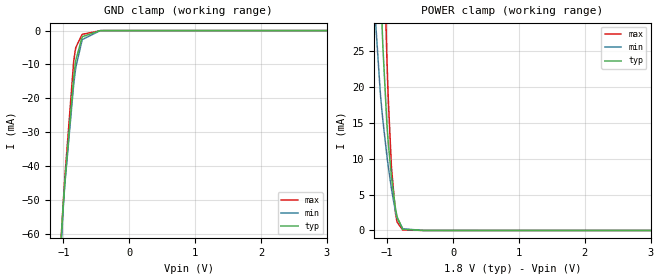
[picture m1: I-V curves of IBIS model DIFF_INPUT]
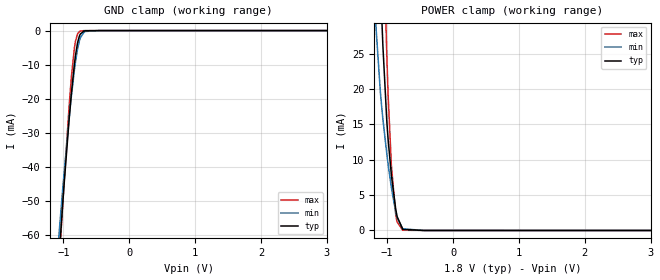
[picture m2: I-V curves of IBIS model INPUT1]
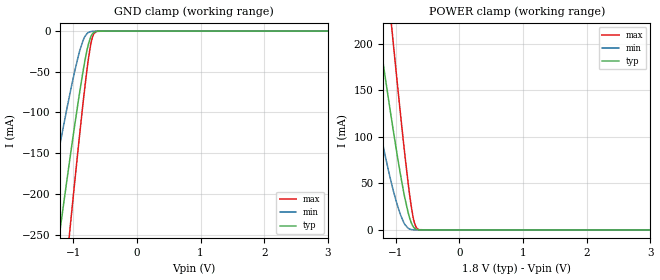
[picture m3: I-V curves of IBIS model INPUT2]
|Texas Instruments Incorporated
|FPD-Link III 4.16 Gbps Serializer w/CSI-2 interface for 2.3MP/60fps cameras
|Marketing part#   Digital Voltage Range   Package-type   #pins
|DS90UB953A-Q1   1.71V to 1.89V   QFN   32
[IBIS Ver]   4.1
[File name]   ds90ub953a-q1.ibs
[File Rev]   1.0
[Date]   03/19/19
[Source]
| Texas Instruments Incorporated.
| Analog-eLab Design Center, HPA
| 12500 TI Blvd
| Dallas, TX -75243
[Notes]   Revision History:
| Rev 1.0: 03/19/19
| - Initial version of the model
| - Model generated from simulations in SPECTRE
| - Model matched to SPICE simulation
| - C_comp although listed in numerical order of value are
|   obtained from varying PVT conditions. For PVT conditions for
|   each specific value refer the buffer description under
|   respective [Model]. IBIS model user is responsible for using
|   appropriate C_comp to simulate for Signal Integrity.
|* EXCEPTION:*
|*  Differential output pins (DIFF_OUT) can operate with bit rate of 4.16Gbps (or 2.08GHz frequency).
|   However, due to IV-VT mismatches >2.2% in SIMDE for higher frequencies,
|   DIFF_OUT IBIS model is generated at frequency of 250MHz or 500Mbps bit rate.
|*  For DIFF_OUT, VT curves were exacted with delay adjustment so that all three corner's
|   rising and falling edges will align around the same time.
|   Also, initial flat response of 170ps has been removed in VT curves (both rising and falling).
|*  INPUT3 IBIS model corresponds to TDI, TCK, TMS pins which are present in design,
|   but not mentioned in the data-sheet.
|*  TDO pin's (present in schematic design) buffer is similar to that of GPIO's.
|   So, for TDO, GPIO model can be used.
[Disclaimer]
| This model is designed as an aid for customers of Texas Instruments.
| TI and its licensors and suppliers make no warranties, either expressed
| or implied, with respect to this  model, including the warranties of
| merchantability or fitness for a particular purpose. The model is
| provided solely on an "as is" basis. The entire risk as to its quality
| and performance is with the customer.
[Copyright]
(C) Copyright 2019 Texas Instruments Incorporated.All rights reserved.
|   DS90UB953A-Q1
[Component]   DS90UB953A-Q1
[Manufacturer]   TI
[Package]   |QFN (32)
|   typ   min   max
R_pkg   0.067   0.027   0.083
L_pkg   0.937nH   0.593nH   1.143nH
C_pkg   0.144pF   0.126pF   0.200pF
[Pin]  signal_name   model_name   R_pin   L_pin   C_pin
1   CSI_D1P   DIFF_INPUT   NA   NA   NA
2   CSI_D1N   DIFF_INPUT   NA   NA   NA
3   CSI_D0P   DIFF_INPUT   NA   NA   NA
4   CSI_D0N   DIFF_INPUT   NA   NA   NA
5   CSI_CLKP   DIFF_INPUT   NA   NA   NA
6   CSI_CLKN   DIFF_INPUT   NA   NA   NA
7   RES0   nc   NA   NA   NA
8   PDB   INPUT1   NA   NA   NA
9   LPF1   nc   NA   NA   NA
10   VDDPLL_CAP   power   NA   NA   NA
11   VDDPLL   power   NA   NA   NA
12   LPF2   nc   NA   NA   NA
13   DOUTN   DIFF_OUT   NA   NA   NA
14   DOUTP   DIFF_OUT   NA   NA   NA
15   VDDRV_CAP   power   NA   NA   NA
16   VDDRV   power   NA   NA   NA
17   GPIO_0   GPIO   NA   NA   NA
18   GPIO_1   GPIO   NA   NA   NA
19   CLK_OUT/IDx   GPIO   NA   NA   NA
20   CLKIN   GPIO   NA   NA   NA
21   MODE   INPUT2   NA   NA   NA
22   RES1   nc   NA   NA   NA
23   I2C_SDA   IO_OPEN_DRAIN   NA   NA   NA
24   I2C_SCL   IO_OPEN_DRAIN   NA   NA   NA
25   VDDD   power   NA   NA   NA
26   VDD_CAP   power   NA   NA   NA
27   GPIO_2   GPIO   NA   NA   NA
28   GPIO_3   GPIO   NA   NA   NA
29   CSI_D3P   DIFF_INPUT   NA   NA   NA
30   CSI_D3N   DIFF_INPUT   NA   NA   NA
31   CSI_D2P   DIFF_INPUT   NA   NA   NA
32   CSI_D2N   DIFF_INPUT   NA   NA   NA
| Models and submodels in the file (7): DIFF_INPUT (Input), INPUT1 (Input), INPUT2 (Input), INPUT3 (Input), GPIO (I/O), IO_OPEN_DRAIN (I/O_open_drain), DIFF_OUT (Output)
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|   DIFF_INPUT Model
[Model]   DIFF_INPUT
Model_type   Input
Vinl = 0.63
Vinh = 1.17
|   typ   min   max
C_comp   0.643pF   0.2943pF   1.006pF
| Where Nom  PVT is Nominal Process, 1.8V, 27C
|   Fast PVT is Strong Process,  1.89V, -40C
|   Slow PVT is Weak Process,   1.71V, 105C
[Model spec]
|subparameter
Vinl   0.63   0.5985   0.6615
Vinh   1.17   1.1115   1.2285
[Voltage Range]   1.8   1.71   1.89
|Junction Temperature
[Temperature Range]   27   105   -40
[Power Clamp Reference]   1.8   1.71   1.89
[GND Clamp Reference]   0   0   0
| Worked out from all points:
|   POWER clamp passes 1 mA (typ) near -0.81 V on its own axis
[GND Clamp]
|   Voltage   I(typ)   I(min)   I(max)
-1.8V     -624.4mA   -649mA     -608.7mA
-1.098V   -81.74mA   -87.49mA   -82.03mA
-1.006V   -52.48mA   -53.16mA   -51.77mA
-979.2mV  -44.98mA   -45.4mA    -43.38mA
-844.2mV  -13.86mA   -15.81mA   -9.084mA
-822.6mV  -10.25mA   -12.35mA   -6.067mA
-811.8mV  -8.685mA   -10.79mA   -4.955mA
-714.6mV  -1.816mA   -2.648mA   -1.108mA
-444.6mV  -17.03uA   -18.94uA   -49.75uA
3.6V      0A         0A         0A
[POWER Clamp]
|   Voltage   I(typ)   I(min)   I(max)
-1.8V     331.9mA    249.9mA    400.2mA
-1.179V   59.49mA    29.36mA    93.17mA
-1.103V   35.12mA    19.01mA    60.1mA
-1.076V   28.11mA    16.31mA    49.14mA
-1.066V   25.62mA    15.32mA    44.93mA
-1.006V   15.06mA    10.52mA    24.47mA
-984.6mV  12.32mA    8.971mA    18.54mA
-936mV    7.498mA    5.817mA    8.867mA
-876.6mV  3.248mA    2.737mA    2.61mA
-849.6mV  1.896mA    1.725mA    1.174mA
-763.2mV  150.9uA    233uA      49.83uA
3.6V      0A         0A         0A
|   INPUT1 Model
[Model]   INPUT1
Model_type   Input
Vinl = 0.63
Vinh = 1.17
|   typ   min   max
C_comp   1.419pF   1.393pF   1.424pF
| Where Nom  PVT is Nominal Process, 1.8V, 27C
|   Fast PVT is Strong Process,  1.89V, -40C
|   Slow PVT is Weak Process,   1.71V, 105C
[Model spec]
|subparameter
Vinl   0.63   0.5985   0.6615
Vinh   1.17   1.1115   1.2285
[Voltage Range]   1.8   1.71   1.89
|Junction Temperature
[Temperature Range]   27   105   -40
[Power Clamp Reference]   1.8   1.71   1.89
[GND Clamp Reference]   0   0   0
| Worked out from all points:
|   GND clamp passes 1 mA (typ) near -0.74 V on its own axis
|   POWER clamp passes 1 mA (typ) near -0.80 V on its own axis
[GND Clamp]
|   Voltage   I(typ)   I(min)   I(max)
-1.8V     -298mA     -267.8mA   -325mA
-1.06V    -64.74mA   -58.15mA   -66.91mA
-1.012V   -51.07mA   -46.73mA   -51.25mA
-914.4mV  -26.27mA   -25.96mA   -22.47mA
-876.6mV  -17.95mA   -18.79mA   -13.12mA
-833.4mV  -9.837mA   -11.56mA   -5.07mA
-817.2mV  -7.329mA   -9.21mA    -3.105mA
-784.8mV  -3.504mA   -5.314mA   -940.8uA
-752.4mV  -1.371mA   -2.661mA   -231.5uA
-666mV    -62.37uA   -251.7uA   -4.974uA
-444.6mV  -453.1nA   -613.8nA   -563.7nA
3.6V      0A         0A         0A
[POWER Clamp]
|   Voltage   I(typ)   I(min)   I(max)
-1.8V     333.1mA    250.9mA    401.5mA
-1.179V   60.1mA     29.95mA    93.71mA
-1.103V   35.67mA    19.51mA    60.56mA
-1.076V   28.64mA    16.77mA    49.57mA
-1.066V   26.14mA    15.76mA    45.35mA
-1.006V   15.49mA    10.85mA    24.82mA
-984.6mV  12.71mA    9.259mA    18.86mA
-936mV    7.769mA    6.018mA    9.098mA
-871.2mV  3.069mA    2.609mA    2.33mA
-849.6mV  1.979mA    1.793mA    1.201mA
-763.2mV  150uA      234.3uA    33.25uA
3.6V      0A         0A         0A
|   INPUT2 Model
[Model]   INPUT2
Model_type   Input
Vinl = 0.63
Vinh = 1.17
|   typ   min   max
C_comp   0.6431pF   0.2942pF   1.006pF
| Where Nom  PVT is Nominal Process, 1.8V, 27C
|   Fast PVT is Strong Process,  1.89V, -40C
|   Slow PVT is Weak Process,   1.71V, 105C
[Model spec]
|subparameter
Vinl   0.63   0.5985   0.6615
Vinh   1.17   1.1115   1.2285
[Voltage Range]   1.8   1.71   1.89
|Junction Temperature
[Temperature Range]   27   105   -40
[Power Clamp Reference]   1.8   1.71   1.89
[GND Clamp Reference]   0   0   0
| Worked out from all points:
|   GND clamp passes 1 mA (typ) near -0.66 V on its own axis
|   POWER clamp passes 1 mA (typ) near -0.68 V on its own axis
[GND Clamp]
|   Voltage   I(typ)   I(min)   I(max)
-1.8V     -599.8mA   -395.9mA   -850.7mA
-1.552V   -446.4mA   -285.2mA   -646.7mA
-1.411V   -363.2mA   -224.7mA   -532.3mA
-1.211V   -247.3mA   -140.7mA   -371mA
-1.103V   -185.9mA   -97.08mA   -284.9mA
-1.039V   -149.8mA   -72.05mA   -234mA
-892.8mV  -72.4mA    -22.93mA   -122.8mA
-822.6mV  -39.35mA   -7.625mA   -72.94mA
-757.8mV  -15.16mA   -1.617mA   -32.51mA
-693mV    -2.804mA   -252.4uA   -6.329mA
-622.8mV  -230.7uA   -31.08uA   -293.8uA
3.6V      0A         0A         0A
[POWER Clamp]
|   Voltage   I(typ)   I(min)   I(max)
-1.8V     468.1mA    304.7mA    745.5mA
-1.476V   311.3mA    186.7mA    511mA
-1.4V     275.2mA    159.9mA    456.6mA
-1.249V   203.6mA    107.5mA    348.7mA
-1.087V   129mA      56.11mA    234.8mA
-1.033V   105mA      41.17mA    197.5mA
-919.8mV  57.62mA    15.51mA    121.3mA
-795.6mV  16.43mA    1.507mA    45.48mA
-714.6mV  2.657mA    152.9uA    10.04mA
-676.8mV  759.9uA    49.85uA    2.69mA
-628.2mV  129.1uA    11.69uA    304.8uA
3.6V      0A         0A         0A
